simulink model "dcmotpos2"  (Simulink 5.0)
settings: Solver=ode45  StartTime=0.0  StopTime=.1  MaxStep=1e-2  RelTol=1e-2

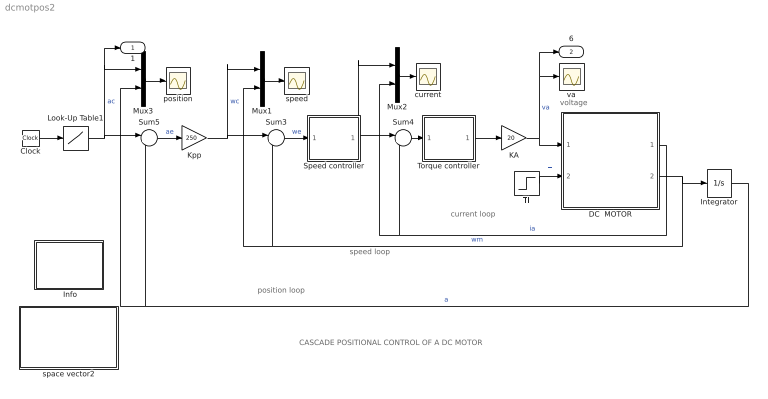
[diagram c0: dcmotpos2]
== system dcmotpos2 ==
  note: voltage
  note: speed loop
  note: current loop
  note: position loop
  note: CASCADE POSITIONAL CONTROL OF A DC MOTOR
  " Info" : Subsystem
  Clock : Clock
  DC  MOTOR : Subsystem  mask{Ra=2.0, La=5.2e-3, J=1.5e-4, Bm=1e-3, K=0.1}
      mask prompts: Ra "Armature resistance [ohm]"; La "Armature inductance [H]"; J "Moment of inertia [Kg.m^2]"; Bm "Frictional torque cefficient"; K "Electromechanical coupling coefficient [N.m/A]"
      mask help: Block diagram of a dc motor with constant fiield excitation.
  Integrator : Integrator
  KA : Gain  Gain=20
  Kpp : Gain  Gain=250
  Look-Up Table1 : Lookup  InputValues="[0  .05  .05 1]"  OutputValues=[1 1 .5 .5 ]
  Mux1 : Mux  Inputs=2
  Mux2 : Mux  Inputs=2
  Mux3 : Mux  Inputs=2
  Speed controller : Subsystem  mask{Kp=1.17, Ki=527, sat=18}
      mask prompts: Kp "Proportional gain (Kp)"; Ki "Integral gain (Ki)"; sat "Saturation limit [pu]"
      mask help: Proportional-Integral Speed Controller
  Sum3 : Sum  Inputs=|+-
  Sum4 : Sum  Inputs=|+-
  Sum5 : Sum  Inputs=|+-
  Tl : Step  Time=0.04  After=0.38  SampleTime=0
  Torque controller : Subsystem  mask{Kp=1.38, Ki=5880, sat=3}
      mask prompts: Kp "Proportional gain (Kp)"; Ki "Integral gain (Ki)"; sat "Saturation limit [pu]"
      mask help: Proportional-Integral Speed Controller
  current : Scope
  position : Scope
  space vector2 : Subsystem
  speed : Scope
  va : Scope
  1 : Outport
  6 : Outport  Port=2
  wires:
  Tl/1 -> DC  MOTOR/2(Tl)  "Tl"
  Mux1/1 -> speed/1
  Mux2/1 -> current/1
  Kpp/1 -> Sum3/1, Mux1/1  "wc"
  DC  MOTOR/1(ia) -> Sum4/2, Mux2/2  "ia"
  Sum5/1 -> Kpp/1  "ae"
  Clock/1 -> Look-Up Table1/1
  Mux3/1 -> position/1
  Look-Up Table1/1 -> Sum5/1, Mux3/1, 1/1  "ac"
  Integrator/1 -> Sum5/2, Mux3/2  "a"
  Speed controller/1(c) -> Sum4/1, Mux2/1
  Sum3/1 -> Speed controller/1(er)  "we"
  Sum4/1 -> Torque controller/1(er)
  Torque controller/1(c) -> KA/1
  KA/1 -> DC  MOTOR/1(va), va/1, 6/1  "va"
  DC  MOTOR/2(wm) -> Integrator/1, Sum3/2, Mux1/2  "wm"

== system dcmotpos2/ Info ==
  note: This demo simulates the cascade position control of a DC motor drive. First, run the model. Second, double click the block.

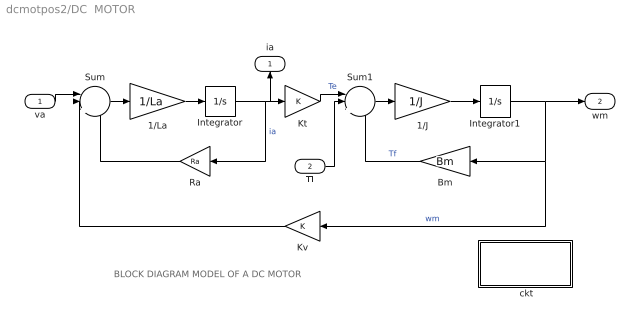
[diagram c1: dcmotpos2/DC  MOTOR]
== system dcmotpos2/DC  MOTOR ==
  note: BLOCK DIAGRAM MODEL OF A DC MOTOR
  va : Inport
  Tl : Inport  Port=2
  " ckt" : Subsystem
  1/J : Gain  Gain=1/J
  1/La : Gain  Gain=1/La
  Bm : Gain  Orientation=left  Gain=Bm
  Integrator : Integrator
  Integrator1 : Integrator
  Kt : Gain  Gain=K
  Kv : Gain  Orientation=left  Gain=K
  Ra : Gain  Orientation=left  Gain=Ra
  Sum : Sum  Inputs=||+--
  Sum1 : Sum  Inputs=||+--
  ia : Outport  Orientation=up
  wm : Outport  Port=2
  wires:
  Kv/1 -> Sum/2
  Ra/1 -> Sum/3
  Kt/1 -> Sum1/1  "Te"
  Bm/1 -> Sum1/3  "Tf"
  Sum/1 -> 1/La/1
  1/La/1 -> Integrator/1
  Integrator/1 -> Ra/1, Kt/1, ia/1  "ia"
  Sum1/1 -> 1/J/1
  1/J/1 -> Integrator1/1
  va/1 -> Sum/1
  Tl/1 -> Sum1/2
  Integrator1/1 -> Bm/1, Kv/1, wm/1  "wm"

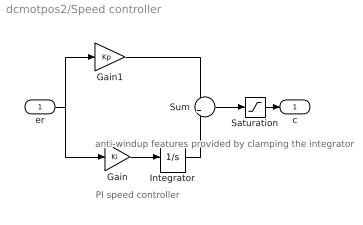
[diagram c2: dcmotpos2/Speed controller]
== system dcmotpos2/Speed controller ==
  note: anti-windup features provided by clamping the integrator
  note: PI speed controller
  er : Inport
  Gain : Gain  Gain=Ki
  Gain1 : Gain  Gain=Kp
  Integrator : Integrator  LimitOutput=on  UpperSaturationLimit=sat  LowerSaturationLimit=-sat
  Saturation : Saturate  UpperLimit=sat  LowerLimit=-sat
  Sum : Sum
  c : Outport  InitialOutput=0
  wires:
  Saturation/1 -> c/1
  Sum/1 -> Saturation/1
  er/1 -> Gain1/1, Gain/1
  Gain1/1 -> Sum/1
  Gain/1 -> Integrator/1
  Integrator/1 -> Sum/2

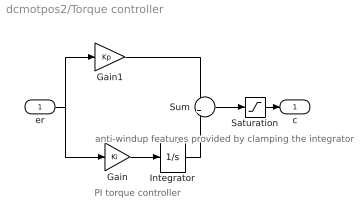
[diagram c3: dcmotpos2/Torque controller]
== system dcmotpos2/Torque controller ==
  note: anti-windup features provided by clamping the integrator
  note: PI torque controller
  er : Inport
  Gain : Gain  Gain=Ki
  Gain1 : Gain  Gain=Kp
  Integrator : Integrator  LimitOutput=on  UpperSaturationLimit=sat  LowerSaturationLimit=-sat
  Saturation : Saturate  UpperLimit=sat  LowerLimit=-sat
  Sum : Sum
  c : Outport  InitialOutput=0
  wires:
  Integrator/1 -> Sum/2
  Gain/1 -> Integrator/1
  Gain1/1 -> Sum/1
  er/1 -> Gain/1, Gain1/1
  Saturation/1 -> c/1
  Sum/1 -> Saturation/1

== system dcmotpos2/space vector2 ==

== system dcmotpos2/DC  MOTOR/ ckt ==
